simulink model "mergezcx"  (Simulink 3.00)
settings: Solver=VariableStepDiscrete  SolverMode=SingleTasking  StartTime=0.0  StopTime=inf  MaxStep=.1  RelTol=1e-3  AbsTol=1e-6
libraries: simulink3 x1

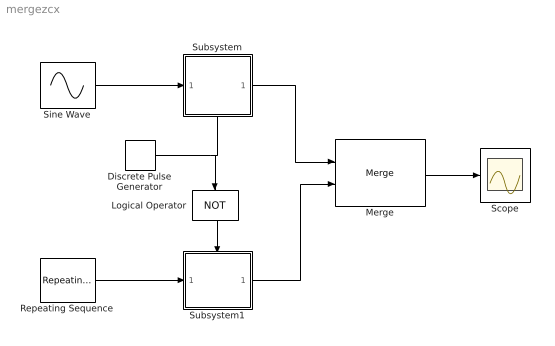
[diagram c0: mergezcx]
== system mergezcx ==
  Discrete Pulse Generator : DiscretePulseGenerator  Amplitude=1  Period=2  PulseWidth=1  PhaseDelay=0  SampleTime=5
  Logical Operator : Logic  Orientation=down  Operator=NOT  Inputs=1
  Merge : Merge  Inputs=2
  Repeating Sequence : simulink3/Sources/Repeating Sequence  rep_seq_t=[0 1]  rep_seq_y=[0 2]
  Scope : Scope
  Sine Wave : Sin  Amplitude=1  Frequency=pi  Phase=0  SampleTime=0
  Subsystem : Subsystem  Tag=MergeExample
  Subsystem1 : Subsystem  Tag=MergeExample
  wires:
  Sine Wave/1 -> Subsystem/1(U)
  Subsystem/1(Y) -> Merge/1
  Subsystem1/1(Y) -> Merge/2
  Logical Operator/1 -> Subsystem1/Enable
  Discrete Pulse Generator/1 -> Logical Operator/1, Subsystem/Enable
  Repeating Sequence/1 -> Subsystem1/1(U)
  Merge/1 -> Scope/1

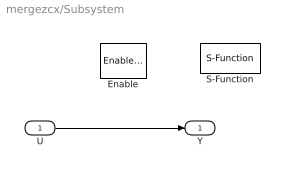
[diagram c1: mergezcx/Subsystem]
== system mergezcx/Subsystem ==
  U : Inport  Port=1  PortWidth=-1  SampleTime=-1  DataType=auto
  Enable : EnablePort  StatesWhenEnabling=reset
  S-Function : S-Function  FunctionName=mergefcn  PortCounts=[]  SFunctionModules=''
  Y : Outport  Port=1
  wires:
  U/1 -> Y/1

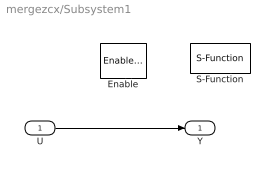
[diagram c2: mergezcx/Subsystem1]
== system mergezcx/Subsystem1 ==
  U : Inport  Port=1  PortWidth=-1  SampleTime=-1  DataType=auto
  Enable : EnablePort  StatesWhenEnabling=reset
  S-Function : S-Function  FunctionName=mergefcn  PortCounts=[]  SFunctionModules=''
  Y : Outport  Port=1
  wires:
  U/1 -> Y/1
